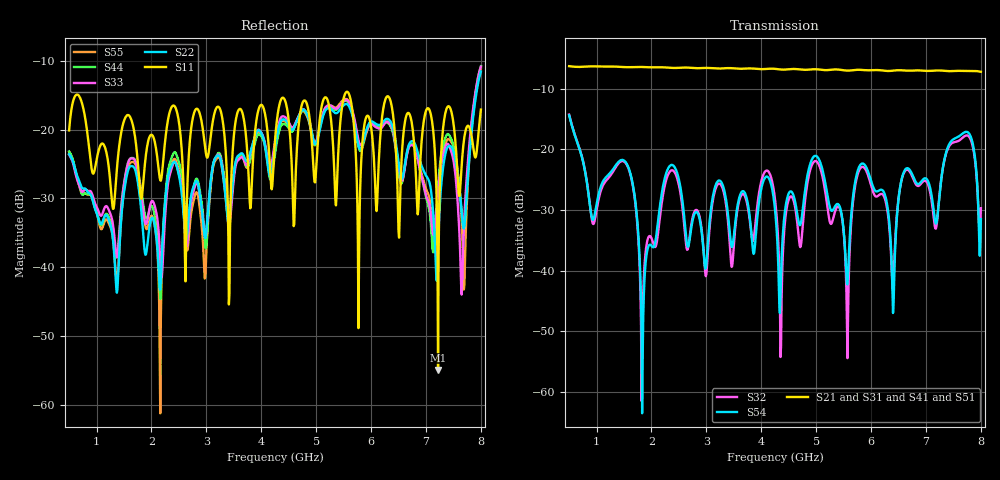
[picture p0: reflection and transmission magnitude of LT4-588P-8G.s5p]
! MTS Systemtechnik GmbH
! S-Parameters
! Model: LT4-588P-8G
! Rohde & Schwarz ZVB8 2Ports - Version 3.20 - 1145.1010k08 SN: 100119
! Converted & adapted with Octave
!		|  MTS  |
!		|  |--o OUT 4 (Port 5)
!		|  |--o OUT 3 (Port 4)
! C (Port 1) o--| LT4-588P-8G |
!  |  |--o OUT 2 (Port 3)
!  |  |--o OUT 1 (Port 2)
! S5P File: Measurements:
! <S11,S12,S13,S14,S15>,
! <S21,S22,S23,S24,S25>,
! <S31,S32,S33,S34,S35>,
! <S41,S42,S43,S44,S45>,
! <S51,S52,S53,S54,S55>:
# HZ  S  DB  R  50.00
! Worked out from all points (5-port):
!   751 points, 500 MHz to 8 GHz, reference 50 ohm
!   strongest paths, dB at 500 MHz, 2.37 GHz, 4.25 GHz, 6.13 GHz, 8 GHz:
!     S21: -6.3, -6.5, -6.7, -6.9, -7.2
!     S31: -6.3, -6.6, -6.7, -7.0, -7.4
!     S41: -6.2, -6.6, -6.8, -7.0, -7.4
!     S51: -6.2, -6.6, -6.8, -7.0, -7.3
!     S54: -14.4, -22.6, -29.9, -26.9, -31.5
!     S32: -14.3, -23.4, -28.2, -27.6, -29.7
!   lowest |S11| = -54.9 dB at 7.22 GHz (marker M1), VSWR 1.00, Z = 49.9 + j0.106 ohm
!   |S11| at or under -10 dB: start of sweep to end of sweep
